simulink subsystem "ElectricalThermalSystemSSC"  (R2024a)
settings: Solver=VariableStepAuto  StartTime=0.0  StopTime=10.0  RelTol=1e-3
undefined symbols (not defined in the file): coolant_pipe_D, coolant_valve_D_ratio_max, coolant_valve_D_ratio_min, coolant_valve_displacement, EnvAirTemp, EnvGrvty, PlantThrEstCmpPwr, PlntThrChArea, PlntThrFanMaxSpd, PlntThrFanMechEff, PlntThrFanVolEff, PlntThrHeaterMaxPwr, PlntThrPipeArea, PlntThrPipeDia, PlntThrPmpMaxSpd, PlntThrRadRamEff, PlntThrRefrigAinit, PlntThrTankArea, PlntThrTankVol, PlntThrValDisp, PlntThrValDratioMax, PlntThrValDratioMin, PlntThrValSplMax, ThrmEM1, ThrmEM2, ThrmEM3, ThrmEM4
libraries: fl_lib x148, nesl_utility x61, SimscapeFluids_lib x25, autolibutils x12
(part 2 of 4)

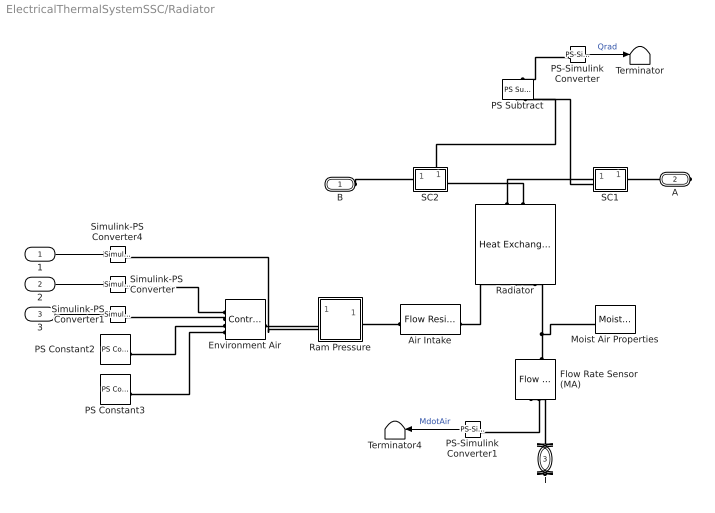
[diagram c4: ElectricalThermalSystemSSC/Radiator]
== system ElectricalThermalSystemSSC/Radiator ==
  1 : Inport
  2 : Inport  Port=2
  3 : Inport  Port=3
  Air Intake : fl_lib/Moist Air/Elements/Flow Resistance (MA)  delta_p_nominal=1e-4 MPa  mdot_nominal=1 kg/s  rho_nominal=1.2 kg/m^3  area=PlntThrRadFanAreaFlw m^2  laminar_fraction=1e-3
  Environment Air : fl_lib/Moist Air/Elements/Controlled Reservoir (MA)  moisture_spec=foundation.enum.moisture_spec.relative_humidity  trace_gas_spec=foundation.enum.trace_gas_spec.mole_fraction  RH_ws=1  area_A=PlntThrRadFanAreaFlw m^2  input_error_spec=foundation.enum.input_range_error.warn
  Flow Rate Sensor (MA) : fl_lib/Moist Air/Sensors/Flow Rate Sensor (MA)  mass_flow_measure=true  volumetric_flow_measure=false  volumetric_flow_conditions=foundation.enum.volumetric_flow_conditions.actual  p_std=0.101325 MPa  T_std=20 degC  RH_std=0.65  energy_flow_measure=true  vapor_flow_measure=false  gas_flow_measure=false
  Moist Air Properties : fl_lib/Moist Air/Utilities/Moist Air Properties (MA)  R_a=287.047 J/kg/K  T_TLU=[-56.55, -50 : 10 : -10, -5 : 1 : 5, 10 : 10 : 350]' degC  h_a_TLU=[342.416126230579; 349.005511058471; 359.063577249119; 369.119948684177; 379.175469465129; 389.230944678417; 394.258910928084; 395.264534937366; 396.27017101329; 397.275819932805; 398.281482472874; 399.287159410541; 400.292851523015; 401.298559587728; 402.304284382408; 403.310026685143; 404.315787274435; 409.34489180313; 419.404921755863; 429.468036401264; 439.535033154839; 449.606720928652; 459.6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  mu_a_TLU=[14.2568883320012; 14.6140127728333; 15.1517277055779; 15.6806860159119; 16.2012351072083; 16.7137043125028; 16.9670071730589; 17.017438062815; 17.0677930842452; 17.1180725309876; 17.1682766951315; 17.2184058672268; 17.2684603362935; 17.3184403898301; 17.3683463138234; 17.4181783927569; 17.4679369096204; 17.7156358640698; 18.2056751785154; 18.68879035749; 19.1652344664982; 19.6352478927873; 20.099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  k_a_TLU=[19.8808489374933; 20.4162454629695; 21.2248743590758; 22.0232452890903; 22.8117314495857; 23.5906913619588; 23.9767075412237; 24.053639990175; 24.1304826682191; 24.2072359051629; 24.2839000294007; 24.3604753679152; 24.4369622462801; 24.5133609886625; 24.5896719178249; 24.6658953551279; 24.7420316205333; 25.1214164701832; 25.8738283029331; 26.6180150229276; 27.3542674377332; 28.0828634735341; 28.8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  p_min=1 kPa  p_max=inf MPa  T_min=-56.55 degC  T_max=350 degC  properties_range_check=simscape.enum.assert.action.error  p_atm=0.101325 MPa  T_atm=20 degC  R_w=461.523 J/kg/K  p_ws_TLU="[1.71168953425982e-06; 3.93770601979424e-06; 1.28411717710344e-05; 3.80051394873809e-05; .00010323902900209; .000259873810798063; .000401741022116384; .000437454836117844; .000476040820618202; .000517704666185737; .000562664883741207; .000611212677444345; .000657088049117899; .000705987905898279; .000758082381149132; .000813549384183233; .000872574861129522; .00122818386934022; .0023392147667769; 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"  h_w_vap_TLU=[2836.88241275372; 2837.81392500514; 2838.63937175807; 2838.7309929628; 2838.06905313927; 2836.62597341095; 2835.60023952573; 2835.37006381376; 2835.13143158077; 2834.88429145066; 2834.62859062897; 2500.93420564316; 2498.55329907119; 2496.17495082036; 2493.79885912205; 2491.42474723191; 2489.05236104642; 2477.20875029194; 2453.54955988604; 2429.83856603313; 2406.00136954922; 2381.97406342174; 2357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  h_w_TLU=[2396.55944251649; 2408.68643343608; 2427.1988031141; 2445.702165897; 2464.18429108356; 2482.62529466839; 2491.82135326629; 2493.6580151792; 2495.49372578218; 2497.32843835745; 2499.16210446923; 2500.99462758899; 2502.83092214066; 2504.6665223621; 2506.50140563013; 2508.335548891; 2510.16892865793; 2519.32352241995; 2537.56068088674; 2555.67742615292; 2573.6403223998; 2591.4109179101; 2608.9455037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  mu_w_TLU=[6.81365662228272; 7.04953750742707; 7.40970098298307; 7.76991278093907; 8.13017290129507; 8.49048134405107; 8.67065368632907; 8.70668960445667; 8.74272600580827; 8.77876289038387; 8.81480025818347; 8.85083810920707; 8.88687644345467; 8.92291526092627; 8.95895456162187; 8.99499434554147; 9.03103461268507; 9.21124319676307; 9.57169660671907; 9.93219833907507; 10.2927483938311; 10.6533467709871; 11.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  k_w_TLU=[11.46288215976; 11.941997488935; 12.676358586935; 13.414208884935; 14.155548382935; 14.900377080935; 15.274099879935; 15.348949115735; 15.423833243535; 15.498752263335; 15.573706175135; 15.648694978935; 15.723718674735; 15.798777262535; 15.873870742335; 15.948999114135; 16.024162377935; 16.400502076935; 17.155798374935; 17.914583872935; 18.676858570935; 19.442622468935; 20.211875566935; 20.984617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  D_w=25 mm^2/s  trace_gas_model=foundation.enum.trace_gas_model.track_fraction  R_g=188.923 J/kg/K  h_g_TLU=[439.555216260064; 444.670268200251; 452.538618847003; 460.487124258496; 468.522588768941; 476.649415958793; 480.74798538725; 481.57054318762; 482.394052398751; 483.218514288831; 484.043930029015; 484.870300696555; 485.697627277859; 486.525910671489; 487.355151691079; 488.185351068185; 489.016509455051; 493.186704139431; 501.599194953048; 510.107689961685; 518.711611080182; 527.410026793075; 536.2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  mu_g_TLU=[10.8921054191698; 11.2215357085649; 11.7233300740382; 12.2234238147811; 12.7215124453467; 13.2173328890673; 13.4643203184773; 13.5136406274989; 13.562934752385; 13.6122025024997; 13.6614436900741; 13.7106581301692; 13.7598456406398; 13.8090060420983; 13.8581391578796; 13.9072448140062; 13.9563228391538; 14.2012926853717; 14.6890687376044; 15.1738428124161; 15.6554929043332; 16.1339159800463; 16.6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  k_g_TLU=[10.489430678843; 10.9507672150864; 11.666197960308; 12.392559739764; 13.1299519771612; 13.8778409888416; 14.2554325416312; 14.3312274189707; 14.4071122346908; 14.4830860227061; 14.5591478179508; 14.6352966574703; 14.7115315815553; 14.787851634907; 14.8642558678259; 14.9407433374142; 15.0173131087819; 15.401364480906; 16.1751373988038; 16.9558134611595; 17.7432208682398; 18.5366976599676; 19.33609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  D_g=16 mm^2/s
  PS Constant2 : fl_lib/Physical Signals/Sources/PS Constant  constant=PlntThrCabRelHInit
  PS Constant3 : fl_lib/Physical Signals/Sources/PS Constant  constant=PlntThrCabCO2Init
  PS Subtract : fl_lib/Physical Signals/Functions/PS Subtract
  PS-Simulink Converter : nesl_utility/PS-Simulink Converter  PhysicalDomain=network_engine_domain  SubClassName=ps_output  LeftPortType=input  RightPortType=output  PseudoPeriodic=off  Frequencies=[]  VectorFormat=inherit  Unit=inherit  AffineConversion=off
  PS-Simulink Converter1 : nesl_utility/PS-Simulink Converter  PhysicalDomain=network_engine_domain  SubClassName=ps_output  LeftPortType=input  RightPortType=output  PseudoPeriodic=off  Frequencies=[]  VectorFormat=inherit  Unit=inherit  AffineConversion=off
  Radiator : SimscapeFluids_lib/Heat Exchangers/Thermal Liquid - Moist Air/Heat Exchanger (TL-MA)  flow_arrangement=fluids.heat_exchangers.enum.FlowArrangementTLMA.Cross  cross_flow_arrangement=fluids.heat_exchangers.enum.CrossFlowArrangementTLMA.MixedUnmixed  R_wall=PlntThrRadThermalR K/W  area_A1=PlntThrPipeArea m^2  area_B1=PlntThrPipeArea m^2  area_A2=PlntThrRadAirAreaFlw m^2  area_B2=PlntThrRadAirAreaFlw m^2  flow_geometry_TL=fluids.heat_exchangers.enum.FlowGeometryTL.InsideTubes  tube_num_TL=PlntThrRadNTubes  tube_length_TL=PlntThrRadLength m  tube_cross_section_TL=fluids.heat_exchangers.enum.TubeCrossSection.Rectangular  tube_diameter_TL=0.1 m  tube_width_TL=PlntThrRadWidth m  tube_height_TL=PlntThrRadTubeHeight m  tube_inner_diameter_TL=0.05 m  tube_outer_diameter_TL=0.1 m  tube_flow_area_TL=0.01 m^2  tube_wetted_perimeter_TL=0.4 m  tube_heat_perimeter_TL=0.4 m  tube_pressure_loss_spec_TL=fluids.heat_exchangers.enum.TubePressureLossSpec.Haaland  tube_loss_coeff_TL=10  tube_local_pressure_loss_spec_TL=fluids.heat_exchangers.enum.LocalLossSpec.AggregateLength  tube_length_add_TL=PlntThrRadTubeLEq m  tube_local_loss_coefficient_TL=0.1  tube_roughness_pressure_TL=15e-6 m  tube_Re_lam_pressure_TL=2000  tube_Re_tur_pressure_TL=4000  tube_shape_factor_generic_TL=64  tube_heat_coeff_spec_TL=fluids.heat_exchangers.enum.TubeHeatCoeffSpec.Gneilinski  tube_colburn_coeff_TL=[.023, .8, .33]  tube_roughness_heat_TL=15e-6 m  tube_Re_lam_heat_TL=2000  tube_Re_tur_heat_TL=4000  tube_Nu_lam_generic_TL=3.66  bank_arrangement_TL=fluids.heat_exchangers.enum.BankArrangement.Inline  bank_num_rows_TL=5  bank_tubes_per_row_TL=5  bank_width_TL=1 m  bank_tube_diameter_TL=0.05 m  bank_longitudinal_pitch_TL=0.15 m  bank_transverse_pitch_TL=0.15 m  bank_pressure_loss_spec_TL=fluids.heat_exchangers.enum.BankPressureLossSpec.Martin  bank_euler_TL=10  bank_heat_coeff_spec_TL=fluids.heat_exchangers.enum.BankHeatCoeffSpec.Martin  bank_colburn_coeff_TL=[.27, .63, .36]  generic_flow_area_TL=0.01 m^2  generic_heat_area_TL=2 m^2  generic_volume_TL=0.05 m^3  generic_loss_coeff_TL=10  generic_colburn_coeff_TL=[.023, .8, .33]  fouling_factor_TL=PltnThrRadCoolFoul m^2*K/kW  fin_area_TL=0 m^2  fin_efficiency_TL=0  p_init_TL=EnvAbsPrs Pa  T_init_TL=EnvAirTemp K  flow_geometry_MA=fluids.heat_exchangers.enum.FlowGeometryMA.Generic  tube_num_MA=1  tube_length_MA=5 m  tube_cross_section_MA=fluids.heat_exchangers.enum.TubeCrossSection.Circular  tube_diameter_MA=0.1 m  tube_width_MA=0.1 m  tube_height_MA=0.1 m  tube_inner_diameter_MA=0.05 m  tube_outer_diameter_MA=0.1 m  tube_flow_area_MA=0.01 m^2  tube_wetted_perimeter_MA=0.4 m  tube_heat_perimeter_MA=0.4 m  tube_pressure_loss_spec_MA=fluids.heat_exchangers.enum.TubePressureLossSpec.Haaland  tube_loss_coeff_MA=10  tube_local_pressure_loss_spec_MA=fluids.heat_exchangers.enum.LocalLossSpec.AggregateLength  tube_length_add_MA=0.1 m  tube_local_loss_coefficient_MA=0.1  tube_roughness_pressure_MA=15e-6 m  tube_Re_lam_pressure_MA=2000  tube_Re_tur_pressure_MA=4000  tube_shape_factor_generic_MA=64  tube_heat_coeff_spec_MA=fluids.heat_exchangers.enum.TubeHeatCoeffSpec.Gneilinski  tube_colburn_coeff_MA=[.023, .8, .33]  tube_roughness_heat_MA=15e-6 m  tube_Re_lam_heat_MA=2000  tube_Re_tur_heat_MA=4000  tube_Nu_lam_generic_MA=3.66  bank_arrangement_MA=fluids.heat_exchangers.enum.BankArrangement.Inline  bank_num_rows_MA=5  bank_tubes_per_row_MA=5  bank_width_MA=1 m  bank_tube_diameter_MA=0.05 m  bank_longitudinal_pitch_MA=0.15 m  bank_transverse_pitch_MA=0.15 m  bank_pressure_loss_spec_MA=fluids.heat_exchangers.enum.BankPressureLossSpec.Martin  bank_euler_MA=10  bank_heat_coeff_spec_MA=fluids.heat_exchangers.enum.BankHeatCoeffSpec.Martin  bank_colburn_coeff_MA=[.27, .63, .36]  generic_flow_area_MA=PlntThrRadAirAreaFlw m^2  generic_heat_area_MA=PlntThrRadAirAreaPr m^2  generic_volume_MA=PlntThrRadMoistAirVol m^3  generic_loss_coeff_MA=10  generic_colburn_coeff_MA=[0.27, 0.63, 0.36]  fouling_factor_MA=PltnThrRadAirFoul m^2*K/kW  fin_area_MA=PlnThrRadAirAreaFins m^2  fin_efficiency_MA=PlntThrRadFinEff  p_init_MA=EnvAbsPrs Pa  T_init_MA=EnvAirTemp K  moisture_spec_MA=foundation.enum.moisture_spec.relative_humidity  RH_init_MA=PlntThrCabRelHInit  x_w_init_MA=0.01  y_w_init_MA=0.01  HR_init_MA=0.01  Tw_init_MA=287 K  trace_gas_spec_MA=foundation.enum.trace_gas_spec.mole_fraction  x_g_init_MA=0.001  y_g_init_MA=PlntThrCabCO2Init  RH_ws_MA=1
  Ram Pressure : Subsystem
  SC1 : Subsystem
  SC2 : Subsystem
  Simulink-PS Converter : nesl_utility/Simulink-PS Converter  PhysicalDomain=network_engine_domain  SubClassName=ps_input  LeftPortType=input  RightPortType=output  PseudoPeriodic=off  Frequencies=[]  NoiseDistribution=none  NoiseParameters=[]  Unit=K  AffineConversion=on  FilteringAndDerivatives=provide  SimscapeFilterOrder=1  InputFilterTimeConstant=0.001  UdotUserProvided=0
  Simulink-PS Converter1 : nesl_utility/Simulink-PS Converter  PhysicalDomain=network_engine_domain  SubClassName=ps_input  LeftPortType=input  RightPortType=output  PseudoPeriodic=off  Frequencies=[]  NoiseDistribution=none  NoiseParameters=[]  Unit=Pa  AffineConversion=off  FilteringAndDerivatives=provide  SimscapeFilterOrder=1  InputFilterTimeConstant=0.001  UdotUserProvided=0
  Simulink-PS Converter4 : nesl_utility/Simulink-PS Converter  PhysicalDomain=network_engine_domain  SubClassName=ps_input  LeftPortType=input  RightPortType=output  PseudoPeriodic=off  Frequencies=[]  NoiseDistribution=none  NoiseParameters=[]  Unit=m/s  AffineConversion=off  FilteringAndDerivatives=provide  SimscapeFilterOrder=1  InputFilterTimeConstant=0.001  UdotUserProvided=0
  Terminator : Terminator
  Terminator4 : Terminator
  B : PMIOPort  Side=Left
  A : PMIOPort  Port=2  Side=Right
  T : PMIOPort  Port=3  Side=Right
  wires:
  3/1 -> Simulink-PS Converter1/1
  2/1 -> Simulink-PS Converter/1
  PS-Simulink Converter/1 -> Terminator/1  "Qrad"
  1/1 -> Simulink-PS Converter4/1
  PS-Simulink Converter1/1 -> Terminator4/1  "MdotAir"
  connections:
  PS-Simulink Converter/LConn1 -- PS Subtract/RConn1
  SC1/LConn2 -- PS Subtract/LConn1
  SC2/LConn2 -- PS Subtract/LConn2
  B/RConn1 -- SC2/LConn1
  Radiator/LConn1 -- SC1/LConn1
  SC1/RConn1 -- A/RConn1
  Radiator/LConn2 -- SC2/RConn1
  Environment Air/RConn2 -- Simulink-PS Converter1/RConn1
  Environment Air/RConn3 -- PS Constant2/RConn1
  Environment Air/RConn4 -- PS Constant3/RConn1
  Environment Air/RConn1 -- Simulink-PS Converter/RConn1
  Flow Rate Sensor (MA)/LConn1 -- Moist Air Properties/RConn1 -- Radiator/RConn1
  Air Intake/RConn1 -- Radiator/RConn2
  Ram Pressure/RConn1 -- Air Intake/LConn1
  Ram Pressure/LConn1 -- Environment Air/LConn1
  Simulink-PS Converter4/RConn1 -- Ram Pressure/LConn2
  T/RConn1 -- Flow Rate Sensor (MA)/RConn1
  Flow Rate Sensor (MA)/RConn2 -- PS-Simulink Converter1/LConn1

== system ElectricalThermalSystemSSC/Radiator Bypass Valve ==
  1 : Inport
  Bias : Bias  Bias=-1
  Flow Resistance (TL) : fl_lib/Thermal Liquid/Elements/Flow Resistance (TL)  delta_p_nominal=0.001 MPa  mdot_nominal=0.3 kg/s  area=pi * PlntThrPipeDia^2 / 4 m^2  laminar_fraction=1e-3
  Gain : Gain  Gain=2
  LPF with IC1 : Subsystem  mask{wc=1, InitCond=0, dataType=off}
      mask prompts: wc "Cutoff frequency, wc [rad/s]"; InitCond "Initial condition, InitCond [same as u]"; dataType "Enforce same input data type"
  Max Valve Displacement [m] : Gain  Gain=PlntThrValDisp
  Radiator Bypass Valve : SimscapeFluids_lib/Thermal Liquid/Valves & Orifices/Directional Control Valves/3-Way Directional Valve (TL)  open_orifices_pos=fluids.thermal_liquid.valves.directional_control_valves.enum.OpenOrifices3Way.PA  open_orifices_neg=fluids.thermal_liquid.valves.directional_control_valves.enum.OpenOrifices3Way.AT  area_spec=fluids.thermal_liquid.valves.directional_control_valves.enum.area_spec.identical  valve_spec=fluids.thermal_liquid.valves.enum.orifice_spec.linear  del_S_max=PlntThrValDisp m  area_max=pi * (PlntThrValDratioMax*PlntThrPipeDia)^2 / 4 m^2  del_S_TLU=[0 0.002 0.004 0.007 0.017] m  valve_area_TLU=[1e-09, 2.0352e-07, 4.0736e-05, .00011438, .00034356] m^2  del_S_flow_TLU=[0 0.002 0.004 0.007 0.017] m  p_diff_TLU=[-.1, .3, .5, .7] MPa  vol_flow_TLU=1e-3 * [1.7e-05, 2e-05, 2.6e-05; .0035, .0045, .0053; .7, .9, 1.06; 1.96, 2.5, 3; 6, 7.7, 9.13] m^3/s  mdot_TLU=[-1e-05, 1.7e-05, 2e-05, 2.6e-05; -.002, .0035, .0045, .0053; -.4, .7, .9, 1.06; -1.13, 1.96, 2.5, 3; -3.45, 6, 7.7, 9.13] kg/s  T_ref_in=293.15 K  p_ref_in=0.101325 MPa  area_leak=pi * (PlntThrValDratioMin*PlntThrPipeDia)^2 / 4 m^2  Cd=0.7  Re_c=12  smoothing_factor=0.01  pressure_recovery=simscape.enum.onoff.on  area=pi * PlntThrPipeDia^2 / 4 m^2  S_max_PA=PlntThrValSplMax m  del_S_max_PA=coolant_valve_displacement-(coolant_valve_displacement)*(pi * (coolant_valve_D_ratio_min*coolant_pipe_D)^2 / 4)/(pi * (coolant_valve_D_ratio_max*coolant_pipe_D)^2 / 4) m  area_max_PA=pi * (coolant_valve_D_ratio_max*coolant_pipe_D)^2 / 4 m^2  del_S_TLU_PA=[0 0.002 0.004 0.007 0.017] m  valve_area_TLU_PA=[1e-09, 2.0352e-07, 4.0736e-05, .00011438, .00034356] m^2  del_S_flow_TLU_PA=[0 0.002 0.004 0.007 0.017] m  p_diff_TLU_PA=[-.1, .3, .5, .7] MPa  vol_flow_TLU_PA=1e-3 * [1.7e-05, 2e-05, 2.6e-05; .0035, .0045, .0053; .7, .9, 1.06; 1.96, 2.5, 3; 6, 7.7, 9.13] m^3/s  mdot_TLU_PA=[-1e-05, 1.7e-05, 2e-05, 2.6e-05; -.002, .0035, .0045, .0053; -.4, .7, .9, 1.06; -1.13, 1.96, 2.5, 3; -3.45, 6, 7.7, 9.13] kg/s  S_max_AT=-PlntThrValSplMax m  del_S_max_AT=coolant_valve_displacement-(coolant_valve_displacement)*(pi * (coolant_valve_D_ratio_min*coolant_pipe_D)^2 / 4)/(pi * (coolant_valve_D_ratio_max*coolant_pipe_D)^2 / 4) m  area_max_AT=pi * (coolant_valve_D_ratio_max*coolant_pipe_D)^2 / 4 m^2  del_S_TLU_AT=[0 0.002 0.004 0.007 0.017] m  valve_area_TLU_AT=[1e-09, 2.0352e-07, 4.0736e-05, .00011438, .00034356] m^2  del_S_flow_TLU_AT=[0 0.002 0.004 0.007 0.017] m  p_diff_TLU_AT=[-.1, .3, .5, .7] MPa  vol_flow_TLU_AT=1e-3 * [1.7e-05, 2e-05, 2.6e-05; .0035, .0045, .0053; .7, .9, 1.06; 1.96, 2.5, 3; 6, 7.7, 9.13] m^3/s  mdot_TLU_AT=[-1e-05, 1.7e-05, 2e-05, 2.6e-05; -.002, .0035, .0045, .0053; -.4, .7, .9, 1.06; -1.13, 1.96, 2.5, 3; -3.45, 6, 7.7, 9.13] kg/s  S_max_PT=2.5e-3 m  del_S_max_PT=0.005 m  area_max_PT=1e-4 m^2  del_S_TLU_PT=[0, .002, .004, .007, .017] m  valve_area_TLU_PT=[1e-09, 2.0352e-07, 4.0736e-05, .00011438, .00034356] m^2  del_S_flow_TLU_PT=[0, .002, .004, .007, .017] m  p_diff_TLU_PT=[.3, .5, .7] MPa  vol_flow_TLU_PT=1e-3 * [1.7e-05, 2e-05, 2.6e-05; .0035, .0045, .0053; .7, .9, 1.06; 1.96, 2.5, 3; 6, 7.7, 9.13] m^3/s  mdot_TLU_PT=[1.7e-05, 2e-05, 2.6e-05; .0035, .0045, .0053; .7, .9, 1.06; 1.96, 2.5, 3; 6, 7.7, 9.13] kg/s
  Simulink-PS Converter : nesl_utility/Simulink-PS Converter  PhysicalDomain=network_engine_domain  SubClassName=ps_input  LeftPortType=input  RightPortType=output  PseudoPeriodic=off  Frequencies=[]  NoiseDistribution=none  NoiseParameters=[]  Unit=m  AffineConversion=off  FilteringAndDerivatives=provide  SimscapeFilterOrder=1  InputFilterTimeConstant=0.001  UdotUserProvided=0
  B : PMIOPort  Side=Left
  C : PMIOPort  Port=2  Side=Left
  A : PMIOPort  Port=3  Side=Right
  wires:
  Max Valve Displacement [m]/1 -> Simulink-PS Converter/1
  Bias/1 -> Max Valve Displacement [m]/1
  Gain/1 -> Bias/1
  1/1 -> LPF with IC1/1(u)
  LPF with IC1/1(y) -> Gain/1
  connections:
  Radiator Bypass Valve/LConn1 -- A/RConn1
  Radiator Bypass Valve/RConn3 -- C/RConn1
  Radiator Bypass Valve/RConn1 -- Simulink-PS Converter/RConn1
  B/RConn1 -- Flow Resistance (TL)/RConn1
  Radiator Bypass Valve/RConn2 -- Flow Resistance (TL)/LConn1

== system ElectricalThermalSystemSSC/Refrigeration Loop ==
  AmbTemp : Inport
  BaroPress : Inport  Port=2
  CmpCmd : Inport  Port=3
  FanCmd : Inport  Port=4
  Power Estimate : Subsystem  VariantControl=Power Estimate
  System Level : Subsystem  VariantControl=System Level
  C : PMIOPort  Side=Left
  T : PMIOPort  Port=2  Side=Left
  D : PMIOPort  Port=3  Side=Right
  CondPress : Outport
  ChlrPress : Outport  Port=2
  CmpPwr : Outport  Port=3
  FanPwr : Outport  Port=4

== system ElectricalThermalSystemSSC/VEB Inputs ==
  VehBody : Inport
  Press : Inport  Port=2
  Temp : Inport  Port=3
  Batt : Inport  Port=4
  LPF with IC1 : Subsystem  mask{wc=100, InitCond=0, dataType=off}
      mask prompts: wc "Cutoff frequency, wc [rad/s]"; InitCond "Initial condition, InitCond [same as u]"; dataType "Enforce same input data type"
  Signal Specification : SignalSpecification  Unit=K
  Terminator : Terminator
  VehicleSpd : Outport
  BaroPress : Outport  Port=2
  AmbTemp : Outport  Port=3
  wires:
  Signal Specification/1 -> AmbTemp/1
  Batt/1 -> Terminator/1
  VehBody/1 -> LPF with IC1/1(u)
  Press/1 -> BaroPress/1
  Temp/1 -> Signal Specification/1
  LPF with IC1/1(y) -> VehicleSpd/1

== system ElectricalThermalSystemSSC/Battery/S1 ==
  Heat Flow Rate Sensor : fl_lib/Thermal/Thermal Sensors/Heat Flow Rate Sensor
  PS-Simulink Converter : nesl_utility/PS-Simulink Converter  PhysicalDomain=network_engine_domain  SubClassName=ps_output  LeftPortType=input  RightPortType=output  PseudoPeriodic=off  Frequencies=[]  VectorFormat=1-D array  Unit=K  AffineConversion=on
  PS-Simulink Converter1 : nesl_utility/PS-Simulink Converter  PhysicalDomain=network_engine_domain  SubClassName=ps_output  LeftPortType=input  RightPortType=output  PseudoPeriodic=off  Frequencies=[]  VectorFormat=inherit  Unit=J/s  AffineConversion=off
  Temperature Sensor : fl_lib/Thermal/Thermal Sensors/Temperature Sensor  temperature_measure=foundation.enum.MeasurementReference.difference
  Terminator : Terminator
  Thermal Reference : fl_lib/Thermal/Thermal Elements/Thermal Reference
  B : PMIOPort  Side=Left
  A : PMIOPort  Port=2  Side=Right
  BattTemp : Outport
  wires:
  PS-Simulink Converter1/1 -> Terminator/1  "QbattSSC"
  PS-Simulink Converter/1 -> BattTemp/1  "BattTempSSC"
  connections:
  Heat Flow Rate Sensor/RConn1 -- PS-Simulink Converter1/LConn1
  Heat Flow Rate Sensor/LConn1 -- Temperature Sensor/LConn1 -- A/RConn1
  Heat Flow Rate Sensor/RConn2 -- B/RConn1
  Thermal Reference/LConn1 -- Temperature Sensor/RConn1
  PS-Simulink Converter/LConn1 -- Temperature Sensor/RConn2

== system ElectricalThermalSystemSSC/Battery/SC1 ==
  Absolute Reference (TL) : fl_lib/Thermal Liquid/Elements/Absolute Reference (TL)
  Mass & Energy Flow Rate Sensor (TL) : fl_lib/Thermal Liquid/Sensors/Flow Rate Sensor (TL)  mass_flow_measure=true  volumetric_flow_measure=false  energy_flow_measure=true
  PS-Simulink Converter : nesl_utility/PS-Simulink Converter  PhysicalDomain=network_engine_domain  SubClassName=ps_output  LeftPortType=input  RightPortType=output  PseudoPeriodic=off  Frequencies=[]  VectorFormat=1-D array  Unit=kg/s  AffineConversion=off
  PS-Simulink Converter1 : nesl_utility/PS-Simulink Converter  PhysicalDomain=network_engine_domain  SubClassName=ps_output  LeftPortType=input  RightPortType=output  PseudoPeriodic=off  Frequencies=[]  VectorFormat=1-D array  Unit=K  AffineConversion=on
  PS-Simulink Converter2 : nesl_utility/PS-Simulink Converter  PhysicalDomain=network_engine_domain  SubClassName=ps_output  LeftPortType=input  RightPortType=output  PseudoPeriodic=off  Frequencies=[]  VectorFormat=inherit  Unit=J/s  AffineConversion=off
  Pressure & Temperature Sensor (TL) : fl_lib/Thermal Liquid/Sensors/Pressure & Temperature Sensor (TL)  reference=foundation.enum.MeasurementReference.difference  pressure=true  pressure_spec=foundation.enum.PressureMeasementSpec.Absolute  temperature=true
  Terminator : Terminator
  Terminator1 : Terminator
  B : PMIOPort  Side=Left
  A : PMIOPort  Port=2  Side=Right
  BattCoolTemp : Outport
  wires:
  PS-Simulink Converter2/1 -> Terminator1/1
  PS-Simulink Converter/1 -> Terminator/1
  PS-Simulink Converter1/1 -> BattCoolTemp/1
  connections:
  PS-Simulink Converter2/LConn1 -- Mass & Energy Flow Rate Sensor (TL)/RConn3
  Pressure & Temperature Sensor (TL)/LConn1 -- A/RConn1 -- Mass & Energy Flow Rate Sensor (TL)/LConn1
  Mass & Energy Flow Rate Sensor (TL)/RConn1 -- B/RConn1
  Absolute Reference (TL)/LConn1 -- Pressure & Temperature Sensor (TL)/RConn1
  PS-Simulink Converter1/LConn1 -- Pressure & Temperature Sensor (TL)/RConn3
  Mass & Energy Flow Rate Sensor (TL)/RConn2 -- PS-Simulink Converter/LConn1

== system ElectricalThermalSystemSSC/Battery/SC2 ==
  Absolute Reference (TL) : fl_lib/Thermal Liquid/Elements/Absolute Reference (TL)
  Mass & Energy Flow Rate Sensor (TL) : fl_lib/Thermal Liquid/Sensors/Flow Rate Sensor (TL)  mass_flow_measure=true  volumetric_flow_measure=false  energy_flow_measure=true
  PS-Simulink Converter : nesl_utility/PS-Simulink Converter  PhysicalDomain=network_engine_domain  SubClassName=ps_output  LeftPortType=input  RightPortType=output  PseudoPeriodic=off  Frequencies=[]  VectorFormat=1-D array  Unit=kg/s  AffineConversion=off
  PS-Simulink Converter1 : nesl_utility/PS-Simulink Converter  PhysicalDomain=network_engine_domain  SubClassName=ps_output  LeftPortType=input  RightPortType=output  PseudoPeriodic=off  Frequencies=[]  VectorFormat=inherit  Unit=J/s  AffineConversion=off
  Pressure & Temperature Sensor (TL) : fl_lib/Thermal Liquid/Sensors/Pressure & Temperature Sensor (TL)  reference=foundation.enum.MeasurementReference.difference  pressure=true  pressure_spec=foundation.enum.PressureMeasementSpec.Absolute  temperature=true
  Terminator : Terminator
  Terminator1 : Terminator
  B : PMIOPort  Side=Left
  A : PMIOPort  Port=2  Side=Right
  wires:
  PS-Simulink Converter1/1 -> Terminator1/1
  PS-Simulink Converter/1 -> Terminator/1
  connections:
  PS-Simulink Converter1/LConn1 -- Mass & Energy Flow Rate Sensor (TL)/RConn3
  Pressure & Temperature Sensor (TL)/LConn1 -- A/RConn1 -- Mass & Energy Flow Rate Sensor (TL)/LConn1
  Mass & Energy Flow Rate Sensor (TL)/RConn1 -- B/RConn1
  Absolute Reference (TL)/LConn1 -- Pressure & Temperature Sensor (TL)/RConn1
  Mass & Energy Flow Rate Sensor (TL)/RConn2 -- PS-Simulink Converter/LConn1

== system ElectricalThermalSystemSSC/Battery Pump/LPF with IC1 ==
  u : Inport
  Cont LPF IC : autolibutils/Cont LPF IC  wc=wc  aMode=1  dataType=off
  Initial Condition : Constant  Value=InitCond  SampleTime=-1
  y : Outport
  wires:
  Initial Condition/1 -> Cont LPF IC/2
  u/1 -> Cont LPF IC/1
  Cont LPF IC/1 -> y/1

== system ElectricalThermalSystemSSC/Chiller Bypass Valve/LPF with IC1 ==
  u : Inport
  Cont LPF IC : autolibutils/Cont LPF IC  wc=wc  aMode=1  dataType=off
  Initial Condition : Constant  Value=InitCond  SampleTime=-1
  y : Outport
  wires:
  Initial Condition/1 -> Cont LPF IC/2
  u/1 -> Cont LPF IC/1
  Cont LPF IC/1 -> y/1

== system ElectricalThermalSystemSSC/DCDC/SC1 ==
  Absolute Reference (TL) : fl_lib/Thermal Liquid/Elements/Absolute Reference (TL)
  Mass & Energy Flow Rate Sensor (TL) : fl_lib/Thermal Liquid/Sensors/Flow Rate Sensor (TL)  mass_flow_measure=true  volumetric_flow_measure=false  energy_flow_measure=true
  PS-Simulink Converter : nesl_utility/PS-Simulink Converter  PhysicalDomain=network_engine_domain  SubClassName=ps_output  LeftPortType=input  RightPortType=output  PseudoPeriodic=off  Frequencies=[]  VectorFormat=1-D array  Unit=W  AffineConversion=off
  PS-Simulink Converter1 : nesl_utility/PS-Simulink Converter  PhysicalDomain=network_engine_domain  SubClassName=ps_output  LeftPortType=input  RightPortType=output  PseudoPeriodic=off  Frequencies=[]  VectorFormat=inherit  Unit=kg/s  AffineConversion=off
  Pressure & Temperature Sensor (TL) : fl_lib/Thermal Liquid/Sensors/Pressure & Temperature Sensor (TL)  reference=foundation.enum.MeasurementReference.difference  pressure=true  pressure_spec=foundation.enum.PressureMeasementSpec.Absolute  temperature=true
  Terminator : Terminator
  Terminator1 : Terminator
  B : PMIOPort  Side=Left
  A : PMIOPort  Port=2  Side=Right
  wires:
  PS-Simulink Converter/1 -> Terminator/1
  PS-Simulink Converter1/1 -> Terminator1/1
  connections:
  Pressure & Temperature Sensor (TL)/LConn1 -- A/RConn1 -- Mass & Energy Flow Rate Sensor (TL)/LConn1
  Mass & Energy Flow Rate Sensor (TL)/RConn1 -- B/RConn1
  Absolute Reference (TL)/LConn1 -- Pressure & Temperature Sensor (TL)/RConn1
  Mass & Energy Flow Rate Sensor (TL)/RConn3 -- PS-Simulink Converter/LConn1
  PS-Simulink Converter1/LConn1 -- Mass & Energy Flow Rate Sensor (TL)/RConn2

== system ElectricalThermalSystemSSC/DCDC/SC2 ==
  Absolute Reference (TL) : fl_lib/Thermal Liquid/Elements/Absolute Reference (TL)
  Mass & Energy Flow Rate Sensor (TL) : fl_lib/Thermal Liquid/Sensors/Flow Rate Sensor (TL)  mass_flow_measure=true  volumetric_flow_measure=false  energy_flow_measure=true
  PS-Simulink Converter : nesl_utility/PS-Simulink Converter  PhysicalDomain=network_engine_domain  SubClassName=ps_output  LeftPortType=input  RightPortType=output  PseudoPeriodic=off  Frequencies=[]  VectorFormat=1-D array  Unit=W  AffineConversion=off
  Pressure & Temperature Sensor (TL) : fl_lib/Thermal Liquid/Sensors/Pressure & Temperature Sensor (TL)  reference=foundation.enum.MeasurementReference.difference  pressure=true  pressure_spec=foundation.enum.PressureMeasementSpec.Absolute  temperature=true
  Terminator : Terminator
  B : PMIOPort  Side=Left
  A : PMIOPort  Port=2  Side=Right
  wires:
  PS-Simulink Converter/1 -> Terminator/1
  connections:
  Pressure & Temperature Sensor (TL)/LConn1 -- A/RConn1 -- Mass & Energy Flow Rate Sensor (TL)/LConn1
  Mass & Energy Flow Rate Sensor (TL)/RConn1 -- B/RConn1
  Absolute Reference (TL)/LConn1 -- Pressure & Temperature Sensor (TL)/RConn1
  Mass & Energy Flow Rate Sensor (TL)/RConn3 -- PS-Simulink Converter/LConn1

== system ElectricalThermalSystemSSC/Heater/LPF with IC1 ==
  u : Inport
  Cont LPF IC : autolibutils/Cont LPF IC  wc=wc  aMode=1  dataType=off
  Initial Condition : Constant  Value=InitCond  SampleTime=-1
  y : Outport
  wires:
  Initial Condition/1 -> Cont LPF IC/2
  u/1 -> Cont LPF IC/1
  Cont LPF IC/1 -> y/1

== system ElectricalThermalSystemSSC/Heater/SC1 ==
  Absolute Reference (TL) : fl_lib/Thermal Liquid/Elements/Absolute Reference (TL)
  Mass & Energy Flow Rate Sensor (TL) : fl_lib/Thermal Liquid/Sensors/Flow Rate Sensor (TL)  mass_flow_measure=true  volumetric_flow_measure=false  energy_flow_measure=true
  PS-Simulink Converter : nesl_utility/PS-Simulink Converter  PhysicalDomain=network_engine_domain  SubClassName=ps_output  LeftPortType=input  RightPortType=output  PseudoPeriodic=off  Frequencies=[]  VectorFormat=1-D array  Unit=W  AffineConversion=off
  PS-Simulink Converter1 : nesl_utility/PS-Simulink Converter  PhysicalDomain=network_engine_domain  SubClassName=ps_output  LeftPortType=input  RightPortType=output  PseudoPeriodic=off  Frequencies=[]  VectorFormat=inherit  Unit=K  AffineConversion=on
  Pressure & Temperature Sensor (TL) : fl_lib/Thermal Liquid/Sensors/Pressure & Temperature Sensor (TL)  reference=foundation.enum.MeasurementReference.difference  pressure=true  pressure_spec=foundation.enum.PressureMeasementSpec.Absolute  temperature=true
  Terminator : Terminator
  Terminator1 : Terminator
  B : PMIOPort  Side=Left
  A : PMIOPort  Port=2  Side=Right
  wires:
  PS-Simulink Converter/1 -> Terminator/1
  PS-Simulink Converter1/1 -> Terminator1/1
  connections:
  Pressure & Temperature Sensor (TL)/LConn1 -- A/RConn1 -- Mass & Energy Flow Rate Sensor (TL)/LConn1
  Mass & Energy Flow Rate Sensor (TL)/RConn1 -- B/RConn1
  Absolute Reference (TL)/LConn1 -- Pressure & Temperature Sensor (TL)/RConn1
  Mass & Energy Flow Rate Sensor (TL)/RConn3 -- PS-Simulink Converter/LConn1
  PS-Simulink Converter1/LConn1 -- Pressure & Temperature Sensor (TL)/RConn3

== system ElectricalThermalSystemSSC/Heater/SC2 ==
  Absolute Reference (TL) : fl_lib/Thermal Liquid/Elements/Absolute Reference (TL)
  Mass & Energy Flow Rate Sensor (TL) : fl_lib/Thermal Liquid/Sensors/Flow Rate Sensor (TL)  mass_flow_measure=true  volumetric_flow_measure=false  energy_flow_measure=true
  PS-Simulink Converter : nesl_utility/PS-Simulink Converter  PhysicalDomain=network_engine_domain  SubClassName=ps_output  LeftPortType=input  RightPortType=output  PseudoPeriodic=off  Frequencies=[]  VectorFormat=1-D array  Unit=W  AffineConversion=off
  Pressure & Temperature Sensor (TL) : fl_lib/Thermal Liquid/Sensors/Pressure & Temperature Sensor (TL)  reference=foundation.enum.MeasurementReference.difference  pressure=true  pressure_spec=foundation.enum.PressureMeasementSpec.Absolute  temperature=true
  Terminator : Terminator
  B : PMIOPort  Side=Left
  A : PMIOPort  Port=2  Side=Right
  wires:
  PS-Simulink Converter/1 -> Terminator/1
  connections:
  Pressure & Temperature Sensor (TL)/LConn1 -- A/RConn1 -- Mass & Energy Flow Rate Sensor (TL)/LConn1
  Mass & Energy Flow Rate Sensor (TL)/RConn1 -- B/RConn1
  Absolute Reference (TL)/LConn1 -- Pressure & Temperature Sensor (TL)/RConn1
  Mass & Energy Flow Rate Sensor (TL)/RConn3 -- PS-Simulink Converter/LConn1

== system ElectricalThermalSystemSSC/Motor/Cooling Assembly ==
  CoolingAssy1 : Subsystem  VariantControl=PlntEMNum == 1
  CoolingAssy2 : Subsystem  VariantControl=PlntEMNum == 2
  CoolingAssy3 : Subsystem  VariantControl=PlntEMNum == 3
  CoolingAssy4 : Subsystem  VariantControl=PlntEMNum == 4
  A : PMIOPort  Side=Left
  B : PMIOPort  Port=2  Side=Right
  H4 : PMIOPort  Port=3  Side=Right
  H3 : PMIOPort  Port=4  Side=Right
  H2 : PMIOPort  Port=5  Side=Right
  H1 : PMIOPort  Port=6  Side=Right
  EMTemp : Outport

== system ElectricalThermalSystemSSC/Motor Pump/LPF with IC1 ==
  u : Inport
  Cont LPF IC : autolibutils/Cont LPF IC  wc=wc  aMode=1  dataType=off
  Initial Condition : Constant  Value=InitCond  SampleTime=-1
  y : Outport
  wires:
  Initial Condition/1 -> Cont LPF IC/2
  u/1 -> Cont LPF IC/1
  Cont LPF IC/1 -> y/1

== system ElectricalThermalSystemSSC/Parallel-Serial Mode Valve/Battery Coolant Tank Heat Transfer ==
  AmbTemp : Inport
  Convective Heat Transfer : fl_lib/Thermal/Thermal Elements/Convective Heat Transfer  thermal_type=foundation.enum.constant_variable.constant  area=3 * PlntThrTankArea m^2  heat_tr_coeff=20 W/(m^2 * K)  min_heat_tr_coeff=1e-3 W/(K*m^2)  T_specify=off  T_priority=None  T=0 K  T_nominal_specify=off  T_nominal_value=1  T_nominal_unit=K  Q_specify=off  Q_priority=None  Q=0 W  Q_nominal_specify=off  Q_nominal_value=1  Q_nominal_unit=W
  Convective Heat Transfer1 : fl_lib/Thermal/Thermal Elements/Convective Heat Transfer  thermal_type=foundation.enum.constant_variable.constant  area=3 * PlntThrTankArea m^2  heat_tr_coeff=20 W/(m^2 * K)  min_heat_tr_coeff=1e-3 W/(K*m^2)  T_specify=off  T_priority=None  T=0 K  T_nominal_specify=off  T_nominal_value=1  T_nominal_unit=K  Q_specify=off  Q_priority=None  Q=0 W  Q_nominal_specify=off  Q_nominal_value=1  Q_nominal_unit=W
  Environment Temperature : fl_lib/Thermal/Thermal Sources/Controlled Temperature Source
  Simulink-PS Converter : nesl_utility/Simulink-PS Converter  PhysicalDomain=network_engine_domain  SubClassName=ps_input  LeftPortType=input  RightPortType=output  PseudoPeriodic=off  Frequencies=[]  NoiseDistribution=none  NoiseParameters=[]  Unit=K  AffineConversion=on  FilteringAndDerivatives=provide  SimscapeFilterOrder=1  InputFilterTimeConstant=0.001  UdotUserProvided=0
  Thermal Reference : fl_lib/Thermal/Thermal Elements/Thermal Reference
  A : PMIOPort  Side=Left
  B : PMIOPort  Port=2  Side=Left
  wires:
  AmbTemp/1 -> Simulink-PS Converter/1
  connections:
  Environment Temperature/LConn1 -- Convective Heat Transfer/RConn1 -- Convective Heat Transfer1/RConn1
  Thermal Reference/LConn1 -- Environment Temperature/RConn2
  Simulink-PS Converter/RConn1 -- Environment Temperature/RConn1
  B/RConn1 -- Convective Heat Transfer1/LConn1
  Convective Heat Transfer/LConn1 -- A/RConn1

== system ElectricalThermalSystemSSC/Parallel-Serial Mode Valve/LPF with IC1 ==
  u : Inport
  Cont LPF IC : autolibutils/Cont LPF IC  wc=wc  aMode=1  dataType=off
  Initial Condition : Constant  Value=InitCond  SampleTime=-1
  y : Outport
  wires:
  Initial Condition/1 -> Cont LPF IC/2
  u/1 -> Cont LPF IC/1
  Cont LPF IC/1 -> y/1

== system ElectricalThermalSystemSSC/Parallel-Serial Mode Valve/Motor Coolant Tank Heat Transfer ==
  AmbTemp : Inport
  Convective Heat Transfer : fl_lib/Thermal/Thermal Elements/Convective Heat Transfer  thermal_type=foundation.enum.constant_variable.constant  area=3 * PlntThrTankArea m^2  heat_tr_coeff=20 W/(m^2 * K)  min_heat_tr_coeff=1e-3 W/(K*m^2)  T_specify=off  T_priority=None  T=0 K  T_nominal_specify=off  T_nominal_value=1  T_nominal_unit=K  Q_specify=off  Q_priority=None  Q=0 W  Q_nominal_specify=off  Q_nominal_value=1  Q_nominal_unit=W
  Convective Heat Transfer1 : fl_lib/Thermal/Thermal Elements/Convective Heat Transfer  thermal_type=foundation.enum.constant_variable.constant  area=3 * PlntThrTankArea m^2  heat_tr_coeff=20 W/(m^2 * K)  min_heat_tr_coeff=1e-3 W/(K*m^2)  T_specify=off  T_priority=None  T=0 K  T_nominal_specify=off  T_nominal_value=1  T_nominal_unit=K  Q_specify=off  Q_priority=None  Q=0 W  Q_nominal_specify=off  Q_nominal_value=1  Q_nominal_unit=W
  Environment Temperature : fl_lib/Thermal/Thermal Sources/Controlled Temperature Source
  Simulink-PS Converter : nesl_utility/Simulink-PS Converter  PhysicalDomain=network_engine_domain  SubClassName=ps_input  LeftPortType=input  RightPortType=output  PseudoPeriodic=off  Frequencies=[]  NoiseDistribution=none  NoiseParameters=[]  Unit=K  AffineConversion=on  FilteringAndDerivatives=provide  SimscapeFilterOrder=1  InputFilterTimeConstant=0.001  UdotUserProvided=0
  Thermal Reference : fl_lib/Thermal/Thermal Elements/Thermal Reference
  A : PMIOPort  Side=Right
  B : PMIOPort  Port=2  Side=Right
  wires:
  AmbTemp/1 -> Simulink-PS Converter/1
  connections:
  Simulink-PS Converter/RConn1 -- Environment Temperature/RConn1
  Thermal Reference/LConn1 -- Environment Temperature/RConn2
  Convective Heat Transfer/RConn1 -- Environment Temperature/LConn1 -- Convective Heat Transfer1/RConn1
  B/RConn1 -- Convective Heat Transfer1/LConn1
  A/RConn1 -- Convective Heat Transfer/LConn1

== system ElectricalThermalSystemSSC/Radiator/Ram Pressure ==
  1/2 : fl_lib/Physical Signals/Functions/PS Gain  gain=0.5
  Controlled Pressure Source (MA) : fl_lib/Moist Air/Sources/Pressure Source (MA)  source_type=foundation.enum.constant_controlled.controlled  pressure_differential=0 MPa  power_spec=foundation.enum.power_spec.isentropic  area_A=PlntThrCabDucArea m^2  area_B=PlntThrCabDucArea m^2
  PS Gain : fl_lib/Physical Signals/Functions/PS Gain  gain=PlntThrRadRamEff
  PS Product : fl_lib/Physical Signals/Functions/PS Product
  Thermodynamic Properties Sensor (MA) : fl_lib/Moist Air/Sensors/Thermodynamic Properties Sensor (MA)  measurement_mass_spec=foundation.enum.measurement_mass_spec.mixture  enthalpy=true  enthalpy_reference=foundation.enum.EnthalpyReference.PropertyTables  density=true  specific_heat=true  entropy=true
  sqr : fl_lib/Physical Signals/Functions/PS Math Function  fcn_choice=foundation.enum.math_function.square  v=1
  A : PMIOPort  Side=Left
  V : PMIOPort  Port=2  Side=Left
  B : PMIOPort  Port=3  Side=Right
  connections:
  PS Gain/RConn1 -- PS Product/LConn1
  Controlled Pressure Source (MA)/RConn1 -- B/RConn1
  Controlled Pressure Source (MA)/LConn1 -- A/RConn1 -- Thermodynamic Properties Sensor (MA)/LConn1
  PS Product/RConn1 -- Controlled Pressure Source (MA)/LConn2
  1/2/RConn1 -- PS Gain/LConn1
  sqr/RConn1 -- 1/2/LConn1
  V/RConn1 -- sqr/LConn1
  Thermodynamic Properties Sensor (MA)/RConn2 -- PS Product/LConn2

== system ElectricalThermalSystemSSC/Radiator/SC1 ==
  Absolute Reference (TL) : fl_lib/Thermal Liquid/Elements/Absolute Reference (TL)
  Mass & Energy Flow Rate Sensor (TL) : fl_lib/Thermal Liquid/Sensors/Flow Rate Sensor (TL)  mass_flow_measure=true  volumetric_flow_measure=false  energy_flow_measure=true
  PS-Simulink Converter1 : nesl_utility/PS-Simulink Converter  PhysicalDomain=network_engine_domain  SubClassName=ps_output  LeftPortType=input  RightPortType=output  PseudoPeriodic=off  Frequencies=[]  VectorFormat=inherit  Unit=K  AffineConversion=on
  Pressure & Temperature Sensor (TL) : fl_lib/Thermal Liquid/Sensors/Pressure & Temperature Sensor (TL)  reference=foundation.enum.MeasurementReference.difference  pressure=true  pressure_spec=foundation.enum.PressureMeasementSpec.Absolute  temperature=true
  Terminator1 : Terminator
  B : PMIOPort  Side=Left
  A : PMIOPort  Port=2  Side=Right
  RadIn : PMIOPort  Port=3  Side=Left
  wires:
  PS-Simulink Converter1/1 -> Terminator1/1
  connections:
  PS-Simulink Converter1/LConn1 -- Pressure & Temperature Sensor (TL)/RConn3
  Pressure & Temperature Sensor (TL)/LConn1 -- A/RConn1 -- Mass & Energy Flow Rate Sensor (TL)/LConn1
  Mass & Energy Flow Rate Sensor (TL)/RConn1 -- B/RConn1
  Absolute Reference (TL)/LConn1 -- Pressure & Temperature Sensor (TL)/RConn1
  RadIn/RConn1 -- Mass & Energy Flow Rate Sensor (TL)/RConn3

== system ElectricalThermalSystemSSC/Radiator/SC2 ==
  Absolute Reference (TL) : fl_lib/Thermal Liquid/Elements/Absolute Reference (TL)
  Mass & Energy Flow Rate Sensor (TL) : fl_lib/Thermal Liquid/Sensors/Flow Rate Sensor (TL)  mass_flow_measure=true  volumetric_flow_measure=false  energy_flow_measure=true
  PS-Simulink Converter1 : nesl_utility/PS-Simulink Converter  PhysicalDomain=network_engine_domain  SubClassName=ps_output  LeftPortType=input  RightPortType=output  PseudoPeriodic=off  Frequencies=[]  VectorFormat=inherit  Unit=K  AffineConversion=on
  Pressure & Temperature Sensor (TL) : fl_lib/Thermal Liquid/Sensors/Pressure & Temperature Sensor (TL)  reference=foundation.enum.MeasurementReference.difference  pressure=true  pressure_spec=foundation.enum.PressureMeasementSpec.Absolute  temperature=true
  Terminator1 : Terminator
  B : PMIOPort  Side=Left
  A : PMIOPort  Port=2  Side=Right
  RadOut : PMIOPort  Port=3  Side=Left
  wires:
  PS-Simulink Converter1/1 -> Terminator1/1
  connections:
  RadOut/RConn1 -- Mass & Energy Flow Rate Sensor (TL)/RConn3
  PS-Simulink Converter1/LConn1 -- Pressure & Temperature Sensor (TL)/RConn3
  Pressure & Temperature Sensor (TL)/LConn1 -- A/RConn1 -- Mass & Energy Flow Rate Sensor (TL)/LConn1
  Mass & Energy Flow Rate Sensor (TL)/RConn1 -- B/RConn1
  Absolute Reference (TL)/LConn1 -- Pressure & Temperature Sensor (TL)/RConn1

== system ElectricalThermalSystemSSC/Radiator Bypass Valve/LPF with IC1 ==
  u : Inport
  Cont LPF IC : autolibutils/Cont LPF IC  wc=wc  aMode=1  dataType=off
  Initial Condition : Constant  Value=InitCond  SampleTime=-1
  y : Outport
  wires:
  Initial Condition/1 -> Cont LPF IC/2
  u/1 -> Cont LPF IC/1
  Cont LPF IC/1 -> y/1

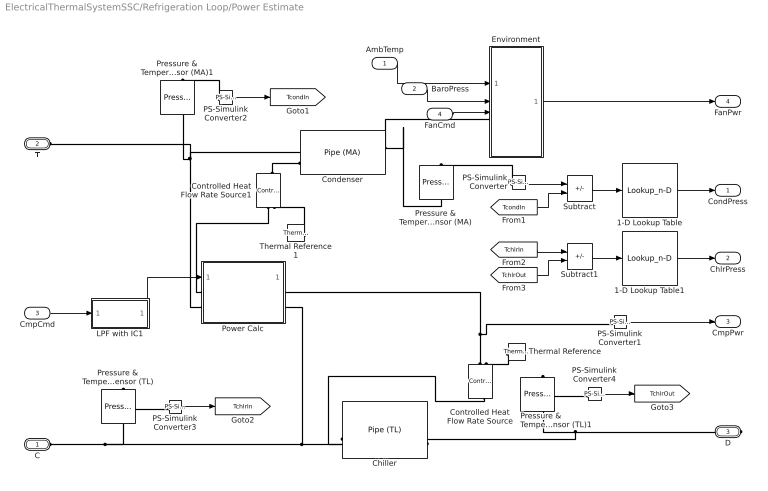
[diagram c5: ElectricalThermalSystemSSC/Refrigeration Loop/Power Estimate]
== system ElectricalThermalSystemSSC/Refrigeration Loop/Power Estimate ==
  AmbTemp : Inport
  BaroPress : Inport  Port=2
  CmpCmd : Inport  Port=3
  FanCmd : Inport  Port=4
  1-D Lookup Table : Lookup_n-D  NumberOfTableDimensions=1  BreakpointsForDimension1=[0 4.5 10 13 20]  Table=[1.3 1.3 1.53 1.62 1.7]  ExtrapMethod=Clip  UseLastTableValue=on  InternalRulePriority=Speed  RndMeth=Simplest
  1-D Lookup Table1 : Lookup_n-D  NumberOfTableDimensions=1  BreakpointsForDimension1=[0 1 3 7]  Table=[0.65 0.45 0.3 0.3]  ExtrapMethod=Clip  UseLastTableValue=on  InternalRulePriority=Speed  RndMeth=Simplest
  Chiller : fl_lib/Thermal Liquid/Elements/Pipe (TL)  length=1 m  area=PlntThrPipeArea m^2  Dh=PlntThrPipeDia m  length_add=0.1 m  roughness=15e-6 m  Re_lam=2000  Re_tur=4000  shape_factor=64  Nu_lam=3.66  dynamic_compressibility=simscape.enum.onoff.on  inertia=simscape.enum.onoff.off  p0=EnvAbsPrs Pa  T0=EnvAirTemp K  mdot0=0 kg/s
  Condenser : fl_lib/Moist Air/Elements/Pipe (MA)  length=0.5 m  area=PlntThrCabDucArea m^2  Dh=PlntThrCabHydDia m  length_add=0 m  roughness=15e-6 m  Re_lam=2000  Re_tur=4000  shape_factor=64  Nu_lam=3.66  wall_condensation=simscape.enum.onoff.off  RH_ws=1  time_constant=1e-3 s  moisture_trace_gas_source=foundation.enum.moisture_trace_gas_source.none  moisture_source_spec=foundation.enum.moisture_source_spec.vapor  moisture_mass_flow=0 kg/s  moisture_temperature_spec=foundation.enum.temperature_spec.atmospheric  moisture_temperature=293.15 K  trace_gas_mass_flow=0 kg/s  trace_gas_temperature_spec=foundation.enum.temperature_spec.atmospheric  trace_gas_temperature=293.15 K  p_I_specify=on  p_I_priority=High  p_I=EnvAbsPrs Pa  p_I_nominal_specify=off  p_I_nominal_value=1  p_I_nominal_unit=MPa  T_I_specify=on  T_I_priority=High  T_I=EnvAirTemp K  T_I_nominal_specify=off  T_I_nominal_value=1  T_I_nominal_unit=K  RH_I_specify=on  RH_I_priority=High  RH_I=PlntThrCabRelHInit  RH_I_nominal_specify=off  RH_I_nominal_value=1  RH_I_nominal_unit=1  x_w_I_specify=off  x_w_I_priority=None  x_w_I=0  x_w_I_nominal_specify=off  x_w_I_nominal_value=1  x_w_I_nominal_unit=1  y_w_I_specify=off  y_w_I_priority=None  y_w_I=0  y_w_I_nominal_specify=off  y_w_I_nominal_value=1  y_w_I_nominal_unit=1  HR_I_specify=off  HR_I_priority=None  HR_I=0  HR_I_nominal_specify=off  HR_I_nominal_value=1  HR_I_nominal_unit=1  x_g_I_specify=on  x_g_I_priority=None  x_g_I=0  x_g_I_nominal_specify=off  x_g_I_nominal_value=1  x_g_I_nominal_unit=1  y_g_I_specify=on  y_g_I_priority=High  y_g_I=PlntThrCabCO2Init  y_g_I_nominal_specify=off  y_g_I_nominal_value=1  y_g_I_nominal_unit=1
  Controlled Heat Flow Rate Source : fl_lib/Thermal/Thermal Sources/Controlled Heat Flow Rate Source
  Controlled Heat Flow Rate Source1 : fl_lib/Thermal/Thermal Sources/Controlled Heat Flow Rate Source
  Environment : Subsystem
  LPF with IC1 : Subsystem  mask{wc=0.2, InitCond=0, dataType=off}
      mask prompts: wc "Cutoff frequency, wc [rad/s]"; InitCond "Initial condition, InitCond [same as u]"; dataType "Enforce same input data type"
  PS-Simulink Converter{,2..4} (4 alike) : nesl_utility/PS-Simulink Converter  PhysicalDomain=network_engine_domain  SubClassName=ps_output  LeftPortType=input  RightPortType=output  PseudoPeriodic=off  Frequencies=[]  VectorFormat=inherit  Unit=inherit  AffineConversion=off
  PS-Simulink Converter1 : nesl_utility/PS-Simulink Converter  PhysicalDomain=network_engine_domain  SubClassName=ps_output  LeftPortType=input  RightPortType=output  PseudoPeriodic=off  Frequencies=[]  VectorFormat=inherit  Unit=W  AffineConversion=off
  Power Calc : Subsystem
  Pressure & Temperature Sensor (MA) : fl_lib/Moist Air/Sensors/Pressure & Temperature Sensor (MA)  reference=foundation.enum.MeasurementReference.absolute  pressure=false  pressure_spec=foundation.enum.PressureMeasementSpec.Absolute  temperature=true
  Pressure & Temperature Sensor (MA)1 : fl_lib/Moist Air/Sensors/Pressure & Temperature Sensor (MA)  reference=foundation.enum.MeasurementReference.absolute  pressure=false  pressure_spec=foundation.enum.PressureMeasementSpec.Absolute  temperature=true
  Pressure & Temperature Sensor (TL) : fl_lib/Thermal Liquid/Sensors/Pressure & Temperature Sensor (TL)  reference=foundation.enum.MeasurementReference.absolute  pressure=false  pressure_spec=foundation.enum.PressureMeasementSpec.Absolute  temperature=true
  Pressure & Temperature Sensor (TL)1 : fl_lib/Thermal Liquid/Sensors/Pressure & Temperature Sensor (TL)  reference=foundation.enum.MeasurementReference.absolute  pressure=false  pressure_spec=foundation.enum.PressureMeasementSpec.Absolute  temperature=true
  Subtract : Sum  Inputs=+-
  Subtract1 : Sum  Inputs=+-
  Thermal Reference : fl_lib/Thermal/Thermal Elements/Thermal Reference
  Thermal Reference1 : fl_lib/Thermal/Thermal Elements/Thermal Reference
  C : PMIOPort  Side=Left
  T : PMIOPort  Port=2  Side=Left
  D : PMIOPort  Port=3  Side=Right
  CondPress : Outport
  ChlrPress : Outport  Port=2
  CmpPwr : Outport  Port=3
  FanPwr : Outport  Port=4
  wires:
  PS-Simulink Converter1/1 -> CmpPwr/1
  Environment/1(FanPwr) -> FanPwr/1
  FanCmd/1 -> Environment/3(FanCmd)
  BaroPress/1 -> Environment/2(BaroPress)
  AmbTemp/1 -> Environment/1(AmbTemp)
  CmpCmd/1 -> LPF with IC1/1(u)
  LPF with IC1/1(y) -> Power Calc/1(Input)
  PS-Simulink Converter4/1 -> [TchlrOut]
  PS-Simulink Converter3/1 -> [TchlrIn]
  PS-Simulink Converter2/1 -> [TcondIn]
  Subtract/1 -> 1-D Lookup Table/1
  Subtract1/1 -> 1-D Lookup Table1/1
  PS-Simulink Converter/1 -> Subtract/1
  [TchlrOut] -> Subtract1/2
  [TcondIn] -> Subtract/2
  [TchlrIn] -> Subtract1/1
  1-D Lookup Table/1 -> CondPress/1
  1-D Lookup Table1/1 -> ChlrPress/1
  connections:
  D/RConn1 -- Pressure & Temperature Sensor (TL)1/LConn1 -- Chiller/RConn1
  Condenser/RConn1 -- Environment/LConn1 -- Pressure & Temperature Sensor (MA)/LConn1
  Power Calc/LConn2 -- Condenser/LConn1 -- T/RConn1 -- Pressure & Temperature Sensor (MA)1/LConn1
  C/RConn1 -- Pressure & Temperature Sensor (TL)/LConn1 -- Chiller/LConn1 -- Power Calc/RConn2
  Controlled Heat Flow Rate Source/LConn1 -- Chiller/LConn2
  Thermal Reference/LConn1 -- Controlled Heat Flow Rate Source/RConn2
  Controlled Heat Flow Rate Source/RConn1 -- Power Calc/RConn1 -- PS-Simulink Converter1/LConn1
  Controlled Heat Flow Rate Source1/RConn1 -- Power Calc/LConn1
  Thermal Reference1/LConn1 -- Controlled Heat Flow Rate Source1/RConn2
  Controlled Heat Flow Rate Source1/LConn1 -- Condenser/LConn2
  Pressure & Temperature Sensor (TL)1/RConn1 -- PS-Simulink Converter4/LConn1
  Pressure & Temperature Sensor (TL)/RConn1 -- PS-Simulink Converter3/LConn1
  PS-Simulink Converter2/LConn1 -- Pressure & Temperature Sensor (MA)1/RConn1
  PS-Simulink Converter/LConn1 -- Pressure & Temperature Sensor (MA)/RConn1
